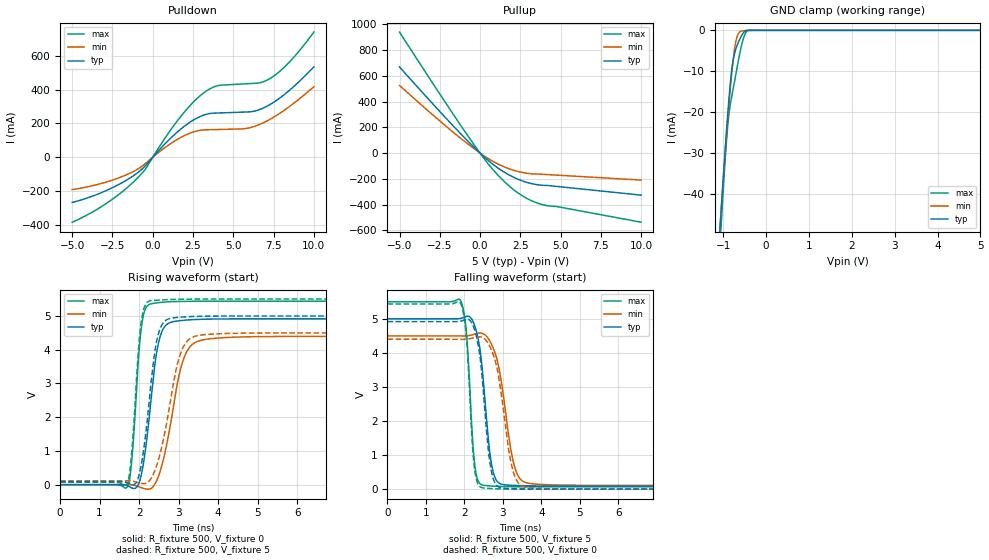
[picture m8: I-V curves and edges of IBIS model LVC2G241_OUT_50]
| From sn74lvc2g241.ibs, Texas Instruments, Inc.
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[Model]   LVC2G241_OUT_50
Model_type  3-state
Enable   Active-High
Vref =   0
Rref =   500
Cref =   50p
Vmeas =   2.5
| variable   typ   min   max
C_comp   5.46pF   4.62pF   6.85pF
| C_pullup   10.66pF   5.37pF   14.35pF
| C_pulldown   8.28pF   6.07pF   11.34pF
| C_tri-state   5.46pF   4.62pF   6.85pF
[Temperature Range]   40   100   -40
| Ambient temperature   25   85   -40
[Voltage range]   5   4.5   5.5
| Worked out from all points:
|   slope of the pulldown table from 0 to 0.75 V, typ, clamps not added: 9.58 ohm
|   slope of the pullup table from 0 to 0.75 V, typ, clamps not added: 9.16 ohm
|   GND clamp passes 1 mA (typ) near -0.56 V on its own axis
|   rising waveform, R_fixture 500, V_fixture 0: 20-80 % time 292ps typ, 430ps min, 187ps max; typ from 0 V to 4.91 V
|   falling waveform, R_fixture 500, V_fixture 5: 20-80 % time 246ps typ, 352ps min, 166ps max; typ from 5 V to 0.09 V
|   rising waveform, R_fixture 500, V_fixture 5: 20-80 % time 289ps typ, 434ps min, 187ps max; typ from 0.09 V to 5 V
|   falling waveform, R_fixture 500, V_fixture 0: 20-80 % time 238ps typ, 341ps min, 163ps max; typ from 4.92 V to 0 V
[GND Clamp]
| LVC2G241_OUT_50
|   Voltage   I(typ)   I(min)   I(max)
-5V       -817.3mA   -761.8mA   -908mA
-1.085V   -50.05mA   -49.49mA   -54.32mA
-1.055V   -45.05mA   -44.88mA   -48.78mA
-905mV    -21.79mA   -23.08mA   -24.44mA
-865mV    -16.46mA   -17.83mA   -20.31mA
-810mV    -10.41mA   -11.29mA   -16.6mA
-765mV    -7.06mA    -6.804mA   -14.06mA
-705mV    -4.512mA   -2.665mA   -10.67mA
-590mV    -1.624mA   -231.7uA   -4.403mA
-505mV    -273.4uA   -88.31uA   -1.237mA
-430mV    -5.996uA   -38.12uA   -30.78uA
5V        30.44pA    126.2nA    731.7pA
[Pulldown]
| LVC2G241_OUT_50
|   Voltage   I(typ)   I(min)   I(max)
-5V       -267.4mA   -191.2mA   -384.4mA
-2.945V   -199.6mA   -148.4mA   -277.3mA
-1.135V   -105.1mA   -81.11mA   -140.5mA
-480mV    -52.75mA   -38.7mA    -73.71mA
1.455V    143.2mA    101.8mA    206.5mA
2.31V     207.2mA    142.6mA    305.4mA
3.085V    246.7mA    161.3mA    375.1mA
4.045V    261.7mA    164.1mA    423.8mA
5.775V    267.7mA    170mA      434.7mA
7.195V    307.4mA    220mA      461.4mA
8.46V     393.8mA    298.3mA    560.8mA
10V       535mA      416.5mA    740.7mA
[Pullup]
| LVC2G241_OUT_50
|   Voltage   I(typ)   I(min)   I(max)
-5V       669.1mA    525.6mA    940mA
-1.98V    253.2mA    194.9mA    360.9mA
45mV      -5.378mA   -4.024mA   -7.822mA
550mV     -61.61mA   -45.63mA   -90.4mA
1.06V     -111mA     -81.25mA   -164.3mA
1.565V    -152.6mA   -110.2mA   -228.1mA
2.07V     -186.9mA   -132.8mA   -282.5mA
2.97V     -230mA     -157.5mA   -356.2mA
3.875V    -250mA     -164.7mA   -400.4mA
4.73V     -258.6mA   -171mA     -414.5mA
10V       -326.7mA   -209.7mA   -536.8mA
[Ramp]
| LVC2G241_OUT_50
| variable   typ   min   max
dV/dt_r   3.02/3.13E-10   2.72/4.49E-10   3.32/1.94E-10
dV/dt_f   2.99/2.57E-10   2.69/3.67E-10   3.31/1.74E-10
R_load = 500
[Rising Waveform]
| LVC2G241_OUT_50
R_fixture =   500
C_fixture =   0
L_fixture =   0
V_fixture =   0
V_fixture_min = 0
V_fixture_max = 0
|   Time   V(typ)   V(min)   V(max)
0s        181.8pV    4.333nV    2.344nV
1.705ns   -33.06mV   5.405mV    -57.95mV
1.82ns    -98.44mV   -5.657mV   813.2mV
2.06ns    320.4mV    -89.79mV   4.694V
2.335ns   2.881V     -83.55mV   5.368V
2.475ns   4.111V     206.9mV    5.391V
2.655ns   4.692V     953.2mV    5.412V
3.12ns    4.87V      3.705V     5.431V
3.68ns    4.904V     4.305V     5.435V
24.99ns   4.914V     4.396V     5.435V
[Falling Waveform]
| LVC2G241_OUT_50
R_fixture =   500
C_fixture =   0
L_fixture =   0
V_fixture =   5
V_fixture_min = 4.5
V_fixture_max = 5.5
|   Time   V(typ)   V(min)   V(max)
0s        5V         4.5V       5.5V
1.91ns    5.016V     4.497V     5.519V
2.055ns   5.069V     4.5V       4.59V
2.27ns    4.798V     4.55V      722.2mV
2.485ns   3.296V     4.564V     114.7mV
2.66ns    1.098V     4.353V     95.65mV
2.81ns    307.5mV    3.953V     84.73mV
3.29ns    111.5mV    728.4mV    73.33mV
3.695ns   97.48mV    166.9mV    71.26mV
24.99ns   89.64mV    109.8mV    70.2mV
[Rising Waveform]
| LVC2G241_OUT_50
R_fixture =   500
C_fixture =   0
L_fixture =   0
V_fixture =   5
V_fixture_min = 4.5
V_fixture_max = 5.5
|   Time   V(typ)   V(min)   V(max)
0s        89.62mV    109.7mV    70.18mV
1.705ns   59.71mV    115mV      44.49mV
1.815ns   8.596mV    105.5mV    996mV
2.04ns    504.1mV    43.16mV    4.705V
2.29ns    2.895V     160.3mV    5.455V
2.435ns   4.2V       534.4mV    5.463V
2.595ns   4.772V     1.235V     5.476V
3.025ns   4.961V     3.802V     5.495V
3.51ns    4.989V     4.425V     5.499V
24.99ns   5V         4.5V       5.5V
[Falling Waveform]
| LVC2G241_OUT_50
R_fixture =   500
C_fixture =   0
L_fixture =   0
V_fixture =   0
V_fixture_min = 0
V_fixture_max = 0
|   Time   V(typ)   V(min)   V(max)
0s        4.917V     4.401V     5.437V
1.905ns   4.932V     4.398V     5.452V
2.05ns    4.979V     4.401V     4.512V
2.26ns    4.704V     4.443V     656mV
2.485ns   2.998V     4.443V     36.31mV
2.64ns    988.5mV    4.241V     22.06mV
2.77ns    251.6mV    3.888V     13.54mV
3.25ns    16.74mV    605.9mV    2.833mV
3.615ns   6.728mV    50.22mV    1.069mV
24.99ns   19.96uV    26.26uV    16.95uV
